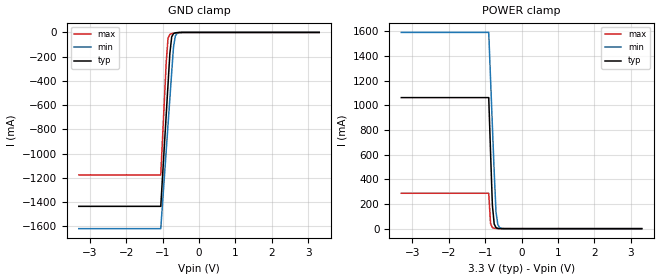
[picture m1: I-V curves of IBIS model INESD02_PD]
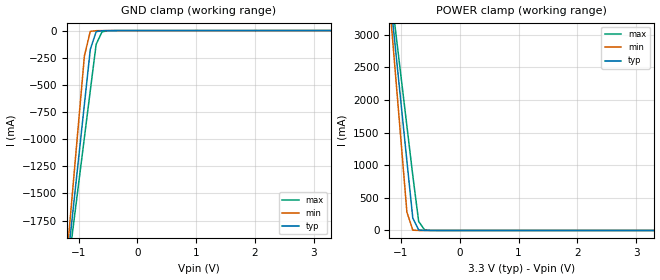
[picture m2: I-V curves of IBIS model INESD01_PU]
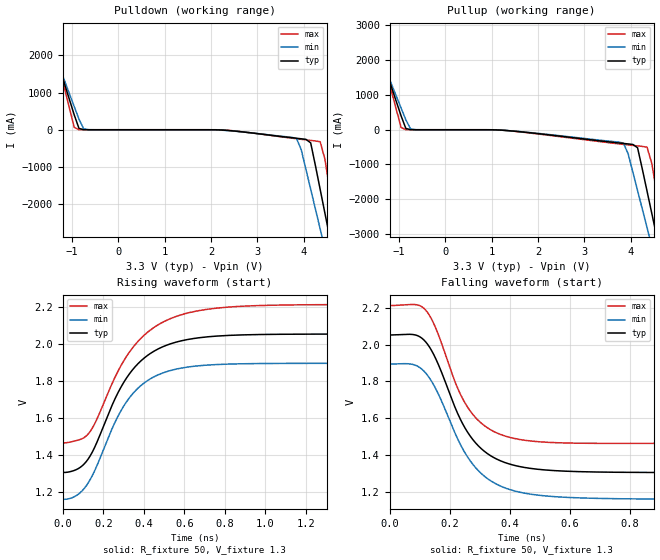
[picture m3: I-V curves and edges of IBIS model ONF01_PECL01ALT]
|   This file is an IBIS representation of the   |
|   Integrated Devices Technology, Inc.   |
|   ICS84330-02   |
|700MHZ, LOW JITTER,CRYSTAL-TO-3.3V DIFFERENTIAL LVPECL FREQUENCY SYNTHESIZER|
[IBIS Ver]   4.1
[File name]   84330_02_3v3.ibs
[File Rev]   1.0
[Date]   31 Dec 2008 | Last modified
|   Apr 20 2005 | Generated
[Source]   Originated at Integrated Devices Technology, Inc.
[Disclaimer]
IDT hereby grants the user of this IBIS model a non-exclusive,
nontransferable license to use this IBIS model under the following terms.
Before using this IBIS model, the user should read this license.
If the user does not accept these terms,  the IBIS model should be
returned to IDT within 30 days.
   The user is granted this license only to use the IBIS model and
is not granted rights to sell, load, rent, lease or license the IBIS
model in whole or in part, or in modified form to anyone other than
user. User may modify the IBIS model to suit its specific
applications but rights to derivative works and such modifications
shall belong to IDT.
   This IBIS model is provided on an "AS IS" basis and IDT makes
absolutely no warranty with respect to the information contained
herein. IDT DISCLAIMS AND CUSTOMER WAIVES ALL WARRANTIES, EXPRESS
OR IMPLIED, INCLUDING WARRANTIES OF MERCHANTABILITY OR FITNESS FOR
A PARTICULAR PURPOSE. The entire risk as to quality and performance
is with the Customer. ACCORDINGLY, IN NO EVENT SHALL THE COMPANY BE
LIABLE FOR ANY DAMAGES, WHETHER IN CONTRACT OR TORT,INCLUDING ANY
LOST PROFITS OR OTHER INCIDENTAL, CONSEQUENTIAL, EXEMPLARY, OR
PUNITIVE DAMAGES ARISING OUT OF THE USE OR APPLICATION OF THE IBIS
model provided in this package. Further, IDT reserves the right to
make changes without notice to any product herein to improve
reliability, function, or design. IDT does not convey any license
under patent rights or any other intellectual property rights,
including those of third parties.
   IDT is not obligated to provide maintenance or support
for the licensed IBIS model.
[Copyright]   Copyright 2005 by Integrated Devices Technology, Inc.
[Component]   ICS84330V-02
[Manufacturer] Integrated Devices Technology, Inc.
[Package]
|PLCC 28 Pin
|   typ   min   max
R_pkg   53.15m   49.2m   57.1m
L_pkg   3.123nH   2.878nH   3.368nH
C_pkg   0.65pF   0.632pF   0.667pF
[Pin] signal_name   model_name   R_pin   L_pin   C_pin
1   VCCA   POWER   49.2m   2.878n   0.632p
2   FREF_EXT   INESD02_PD   51.2m   3.038n   0.643p
3   XTAL_SEL   INESD01_PU   53.8m   3.201n   0.655p
4   XTAL_IN   NC   57.1m   3.368n   0.667p
5   XTAL_OUT   NC   57.1m   3.368n   0.667p
6   OE   INESD01_PU   53.8m   3.201n   0.655p
7   nP_LOAD   INESD01_PU   51.2m   3.038n   0.643p
8   M0   INESD01_PU   49.2m   2.878n   0.632p
9   M1   INESD01_PU   51.2m   3.038n   0.643p
10   M2   INESD01_PU   53.8m   3.201n   0.655p
11   M3   INESD01_PU   57.1m   3.368n   0.667p
12   M4   INESD01_PU   57.1m   3.368n   0.667p
13   M5   INESD01_PU   53.8m   3.201n   0.655p
14   M6   INESD01_PU   51.2m   3.038n   0.643p
15   M7   INESD01_PU   49.2m   2.878n   0.632p
16   M8   INESD01_PU   51.2m   3.038n   0.643p
17   N0   INESD01_PU   53.8m   3.201n   0.655p
18   N1   INESD01_PU   57.1m   3.368n   0.667p
19   VEE   GND   57.1m   3.368n   0.667p
20   TEST   ONF01_PECL01ALT   53.8m   3.201n   0.655p
21   VCC   POWER   51.2m   3.038n   0.643p
22   VEE   GND   49.2m   2.878n   0.632p
23   nFOUT   ONF01_PECL01ALT   51.2m   3.038n   0.643p
24   FOUT   ONF01_PECL01ALT   53.8m   3.201n   0.655p
25   VCC   POWER   57.1m   3.368n   0.667p
26   S_CLOCK   INESD01_PD   57.1m   3.368n   0.667p
27   S_DATA   INESD01_PD   53.8m   3.201n   0.655p
28   S_LOAD   INESD01_PD   51.2m   3.038n   0.643p
[Diff Pin]  inv_pin  vdiff tdelay_typ tdelay_min  tdelay_max
24   23   NA   0  0  0
| Models and submodels in the file (4): INESD02_PD (Input), INESD01_PU (Input), ONF01_PECL01ALT (Output_ECL), INESD01_PD (Input)
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[Model]   INESD02_PD
Model_type   Input
Polarity   Non-Inverting
Vinl = 0.80V
Vinh = 2.0V
|   typ   min   max
C_comp   2pF   1.5pF   2.5pF
|   typ   min   max
[Voltage range]  3.3V   3.15V   3.45V
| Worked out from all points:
|   GND clamp passes 1 mA (typ) near -0.56 V on its own axis
|   POWER clamp passes 1 mA (typ) near -0.61 V on its own axis
[GND_clamp]
|Voltage   I(typ)   I(min)   I(max)
-3.3V     -1.436A    -1.62A     -1.176A
-1.05V    -1.436A    -1.62A     -1.176A
-900mV    -678.5mA   -975.1mA   -244mA
-850mV    -426.1mA   -760.1mA   -46.85mA
-800mV    -173.9mA   -545.4mA   -16.11mA
-750mV    -36.96mA   -330.7mA   -9.916mA
-700mV    -9.696mA   -120.2mA   -7.056mA
-650mV    -3.545mA   -29.7mA    -4.857mA
-600mV    -1.629mA   -7.52mA    -3.049mA
-400mV    -52.81uA   -52.52uA   -108.7uA
3.3V      71.13uA    77.43uA    62.11uA
[POWER_clamp]
|Voltage   I(typ)   I(min)   I(max)
-3.3V     1.063A     1.593A     287.3mA
-900mV    1.063A     1.593A     287.3mA
-850mV    620.5mA    1.215A     41.84mA
-800mV    191.6mA    837.5mA    8.757mA
-750mV    37.76mA    460.2mA    3.328mA
-700mV    8.104mA    133.8mA    1.728mA
-650mV    2.076mA    32.66mA    905.3uA
-600mV    678.1uA    8.083mA    443.8uA
-450mV    104.2uA    213.3uA    89.09uA
3.3V      -3.041nA   -3.986uA   0A
[Model]   INESD01_PU
Model_type   Input
Polarity   Non-Inverting
Vinl = 0.8V
Vinh = 2.0V
|   typ   min   max
C_comp   2pF   1.5pF   2.5pF
|   typ   min   max
[Voltage range]  3.3V   3.15V   3.45V
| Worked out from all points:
|   GND clamp passes 1 mA (typ) near -0.55 V on its own axis
|   POWER clamp passes 1 mA (typ) near -0.61 V on its own axis
[GND_clamp]
|Voltage   I(typ)   I(min)   I(max)
-3.3V     -12.83A    -15.14A    -11.37A
-1.2V     -2.195A    -2.092A    -2.281A
-1.1V     -1.689A    -1.472A    -1.849A
-900mV    -678.5mA   -232.7mA   -984.8mA
-800mV    -174mA     -7.237mA   -553.3mA
-700mV    -9.767mA   -1.114mA   -126.1mA
-600mV    -1.7mA     -240.1uA   -11.15mA
-300mV    -81.66uA   -67.79uA   -163.4uA
3.3V      1.866nA    1.113pA    239.1nA
[POWER_clamp]
|Voltage   I(typ)   I(min)   I(max)
-3.3V     22.38A     26.45A     19.82A
-1.2V     3.723A     3.545A     3.874A
-1.1V     2.836A     2.457A     3.116A
-1V       1.949A     1.369A     2.358A
-900mV    1.063A     281mA      1.601A
-800mV    191.5mA    5.012mA    843.9mA
-700mV    8.032mA    142.2uA    138.3mA
-600mV    607uA      17.63uA    10.62mA
-400mV    16.32uA    7.545uA    335.9uA
3.3V      -71.13uA   -62.11uA   -78.26uA
[Model]   ONF01_PECL01ALT
Model_type  Output_ECL
Polarity   Non-Inverting
Vmeas = 1.636
Rref = 50
Cref = 0
Vref = 1.3
|Variable  typ   min   max
C_comp   2p   1.5p   2.5p
[Voltage Range]   3.3   3.135   3.465
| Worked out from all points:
|   rising waveform, R_fixture 50, V_fixture 1.3: 20-80 % time 218ps typ, 206ps min, 242ps max; typ from 1.31 V to 2.05 V
|   falling waveform, R_fixture 50, V_fixture 1.3: 20-80 % time 134ps typ, 143ps min, 120ps max; typ from 2.05 V to 1.31 V
| Open source, no load
|  Voltage   I(typ)   I(min)   I(max)
[Pullup]
-3.3V     9.786A     8.45A      12.03A
-1.667V   3.247A     2.997A     3.691A
-1.565V   2.839A     2.657A     3.17A
-952.6mV  398mA      622.1mA    64.71mA
-850.5mV  36.63mA    284.2mA    1.532mA
-646.4mV  229.3uA    1.611mA    19.07uA
3.844V    -394.4mA   -383.6mA   -421.3mA
4.151V    -517.8mA   -1.749A    -465.4mA
4.355V    -1.764A    -2.812A    -500.3mA
4.559V    -3.036A    -3.875A    -1.773A
4.763V    -4.308A    -4.937A    -3.393A
6.6V      -15.79A    -14.52A    -18.03A
[Pulldown]
-3.3V     9.786A     8.45A      12.03A
-1.565V   2.839A     2.657A     3.17A
-1.463V   2.432A     2.317A     2.65A
-952.6mV  398mA      622.1mA    64.71mA
-850.5mV  36.63mA    284.2mA    1.532mA
-646.4mV  229.3uA    1.611mA    19.07uA
3.844V    -229.1mA   -232.1mA   -241.8mA
4.151V    -352.7mA   -1.598A    -286.7mA
4.355V    -1.599A    -2.66A     -322.1mA
4.559V    -2.871A    -3.722A    -1.595A
4.763V    -4.144A    -4.785A    -3.217A
6.6V      -15.69A    -14.41A    -17.97A
[Ramp]
|   typ   min   max
dV/dt_r   0.45V/0.37ns   0.45V/0.405ns   0.45V/0.27ns
dV/dt_f   0.45V/0.37ns   0.45V/0.405ns   0.45V/0.27ns
R_load =   50.0000
[Rising Waveform]
R_fixture = 50
V_fixture = 1.3   | VCC_typ - 2V
V_fixture_max = 1.465   | VCC_max - 2V
V_fixture_min = 1.135   | VCC_min - 2V
C_fixture = 0.0p
| Time   typ   min   max
0s        1.306V     1.161V     1.465V
70ps      1.323V     1.183V     1.479V
128ps     1.383V     1.254V     1.517V
258ps     1.703V     1.577V     1.819V
316ps     1.817V     1.689V     1.934V
398ps     1.919V     1.785V     2.042V
504ps     1.988V     1.846V     2.121V
658ps     2.03V      1.879V     2.175V
875ps     2.047V     1.891V     2.201V
2ns       2.052V     1.894V     2.211V
[Falling Waveform]
R_fixture = 50
V_fixture = 1.3   | VCC_typ - 2V
V_fixture_max = 1.465   | VCC_max - 2V
V_fixture_min = 1.135   | VCC_min - 2V
C_fixture = 0.0p
0s        2.052V     1.894V     2.211V
76ps      2.055V     1.893V     2.217V
118ps     2.018V     1.85V      2.19V
150ps     1.936V     1.772V     2.103V
222ps     1.644V     1.505V     1.782V
264ps     1.514V     1.38V      1.65V
326ps     1.409V     1.274V     1.549V
410ps     1.348V     1.21V      1.493V
708ps     1.309V     1.166V     1.465V
2ns       1.306V     1.161V     1.465V
